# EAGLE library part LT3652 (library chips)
Solar power tracking 2A battery charger
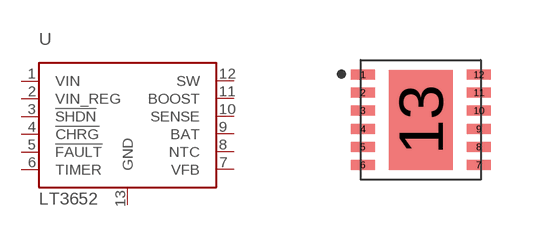
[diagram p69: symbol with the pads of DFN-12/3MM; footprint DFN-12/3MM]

Designator prefix U

## LT3652 (DIGIKEY: LT3652EDD#PBF-ND)  [DFN-12/3MM]
1  VIN
2  VIN_REG
3  !SHDN
4  !CHRG
5  !FAULT
6  TIMER
7  VFB
8  NTC
9  BAT
10  SENSE
11  BOOST
12  SW
13  GND

## Footprint DFN-12/3MM (pad centres in mm)
DFN-12/3MM for FTDI234XD
smd 0.6 x 0.25: 1 -1.45,1.13; 2 -1.45,0.68; 3 -1.45,0.23; 4 -1.45,-0.23; 5 -1.45,-0.68; 6 -1.45,-1.13; 7 1.45,-1.13; 8 1.45,-0.68; 9 1.45,-0.23; 10 1.45,0.23; 11 1.45,0.68; 12 1.45,1.13
smd 1.6 x 2.5: 13 0,0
